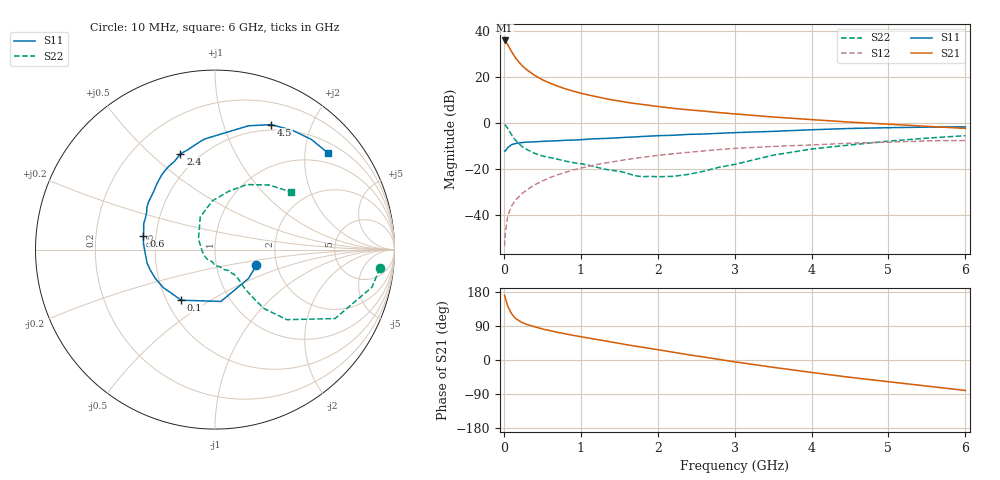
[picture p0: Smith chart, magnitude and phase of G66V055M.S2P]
! SIEMENS Small Signal Semiconductors
! BFG193
! Si NPN RF Bipolar Junction Transistor in SOT223
! VCE = 6 V  IC = 55 mA
! Common Emitter S-Parameters:  August  1996
# GHz  S  MA  R  50
!  f  S11  S21  S12  S22
! GHz  MAG  ANG  MAG  ANG  MAG  ANG  MAG  ANG
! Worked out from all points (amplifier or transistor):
!   36 points, 10 MHz to 6 GHz, reference 50 ohm
!   highest |S21| = 35.9 dB at 10 MHz (marker M1)
!   |S21| within 3 dB of that: start of sweep to 69.67 MHz
!   unconditionally stable (mu >= 1): 452.1 MHz to 2.356 GHz
!   at 250 MHz: K = 0.91, MSG = 27.4 dB, |S12| = -30.3 dB
!   at 1.4 GHz: K = 1.04, MAG = 12.2 dB, |S12| = -16.9 dB
!   at 6 GHz: K = 0.89, MSG = 2.6 dB, |S12| = -7.6 dB
!   S11 on the Smith chart (normalised r, x): 10 MHz: 1.57, -0.29; 100 MHz: 0.59, -0.38; 600 MHz: 0.43, +0.08; 2.4 GHz: 0.40, +0.62; 4.5 GHz: 0.44, +1.45; 6 GHz: 0.74, +2.52
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0.01  0.2466 -20.4  62.59 170.7  0.0021 90.5  0.9248 -6.5
0.02  0.2463 -40.8  60.43 163.1  0.0041 81.1  0.899 -13.5
0.05  0.2906 -83.5  50.79 142.2  0.0095 71.1  0.7708 -29.9
0.1  0.3389 -123.7  35.91 122.3  0.0157 68.0  0.5589 -44.3
0.15  0.3578 -143.9  26.35 110.0  0.0207 66.6  0.4257 -50.3
0.2  0.3696 -154.5  20.77 103.2  0.0256 68.8  0.3509 -51.5
0.25  0.3787 -162.7  16.93 97.8  0.0305 69.1  0.2961 -52.3
0.3  0.3857 -168.9  14.34 93.8  0.0353 69.4  0.2649 -52.5
0.4  0.39 -177.5  10.92 87.8  0.0453 69.8  0.2193 -51.8
0.5  0.4002 175.0  8.769 82.0  0.0549 68.8  0.193 -51.3
0.6  0.4061 169.4  7.374 77.5  0.065 67.7  0.1772 -52.2
0.7  0.4121 164.6  6.35 73.0  0.075 66.4  0.1631 -54.2
0.8  0.4225 160.2  5.549 69.0  0.0847 64.2  0.1487 -56.0
1.1  0.4472 148.0  4.074 58.0  0.1144 59.4  0.1213 -65.8
1.3  0.4614 140.8  3.461 50.9  0.1335 55.3  0.1002 -73.4
1.6  0.4911 130.8  2.819 40.2  0.1615 48.5  0.0814 -93.7
2.2  0.5421 114.4  2.094 20.6  0.2148 35.0  0.0693 -156.8
2.4  0.5671 109.9  1.941 13.8  0.2313 30.8  0.0765 175.2
3.5  0.66 83.6  1.354 -19.3  0.3103 3.9  0.2001 114.2
4.5  0.7631 65.9  1.048 -45.7  0.3652 -16.2  0.334 76.7
5.5  0.8156 48.8  0.85 -68.8  0.4104 -39.4  0.4697 50.0
6  0.8278 40.6  0.766 -80.4  0.4167 -52.8  0.5314 37.2
